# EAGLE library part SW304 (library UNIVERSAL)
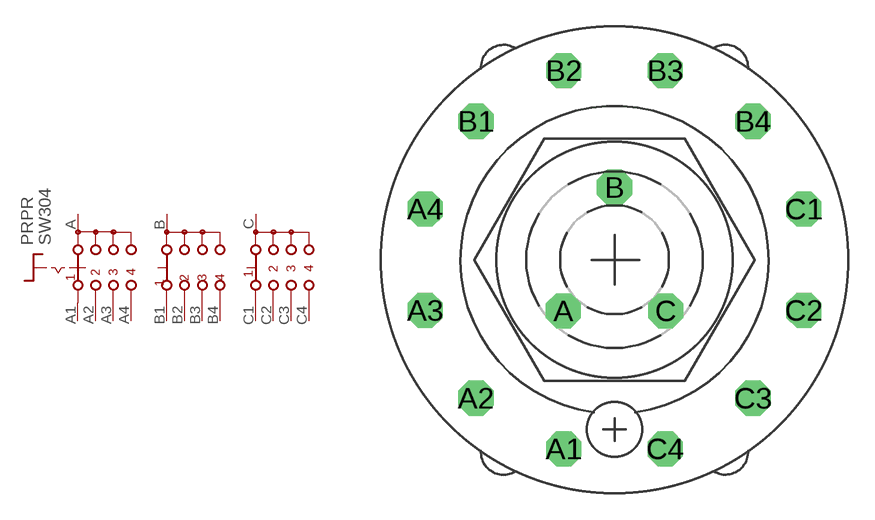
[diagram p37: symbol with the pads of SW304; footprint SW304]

Designator prefix PR; gates PR=SW304A G$2=SW304B G$3=SW304C

## SW304  [SW304]
A  PR:A  pas
A1  PR:A1  pas
A2  PR:A2  pas
A3  PR:A3  pas
A4  PR:A4  pas
B  G$2:B  pas
B1  G$2:B1  pas
B2  G$2:B2  pas
B3  G$2:B3  pas
B4  G$2:B4  pas
C  G$3:C  pas
C1  G$3:C1  pas
C2  G$3:C2  pas
C3  G$3:C3  pas
C4  G$3:C4  pas

## Footprint SW304 (pad centres in mm)
drill 1.321 octagon: A -2.87,-2.87; A1 -2.845,-10.617; A2 -7.772,-7.772; A3 -10.617,-2.845; A4 -10.617,2.845; B 0,4.059; B1 -7.772,7.772; B2 -2.845,10.617; B3 2.845,10.617; B4 7.772,7.772; C 2.87,-2.87; C1 10.617,2.845; C2 10.617,-2.845; C3 7.772,-7.772; C4 2.845,-10.617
